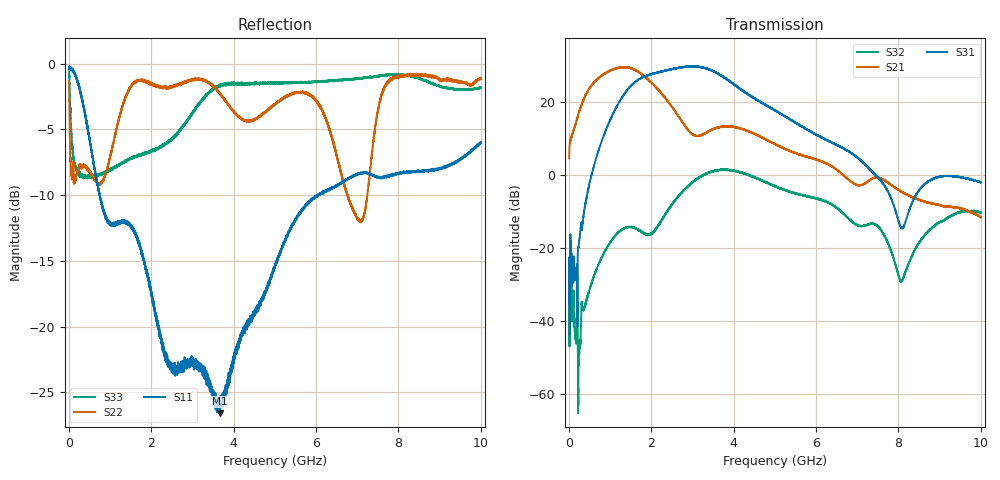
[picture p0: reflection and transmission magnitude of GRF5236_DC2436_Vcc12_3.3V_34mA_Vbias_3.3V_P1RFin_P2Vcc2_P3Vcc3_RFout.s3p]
!Keysight Technologies,N5245B,MY56052315,A.20.20.05
!Date: Friday, August 21, 2026 13:52:32
!Correction: S11(C  3-Port  )
!S12(C  3-Port  )
!S13(C  3-Port  )
!S21(C  3-Port  )
!S22(C  3-Port  )
!S23(C  3-Port  )
!S31(C  3-Port  )
!S32(C  3-Port  )
!S33(C  3-Port  )
!S3P File: Measurements: <S11,S12,S13>,
!<S21,S22,S23>,
!<S31,S32,S33>:
# Hz S  RI  R 50
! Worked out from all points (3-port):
!   9991 points, 10 MHz to 10 GHz, reference 50 ohm
!   strongest paths, dB at 10 MHz, 2.507 GHz, 5.005 GHz, 7.503 GHz, 10 GHz:
!     S31: -29.2, 29.0, 17.7, -0.8, -2.0
!     S21: 4.6, 18.6, 8.4, -0.7, -11.6
!     S32: -34.5, -8.1, -3.0, -14.1, -10.4
!   lowest |S11| = -26.6 dB at 3.659 GHz (marker M1), VSWR 1.10, Z = 51.8 + j4.4 ohm
!   |S11| at or under -10 dB: 749.2 MHz to 6.039 GHz (5.289 GHz wide, 156 % of centre); 6.039756 GHz to 6.042862 GHz (3.106 MHz wide, 0.0514 % of centre); 6.052386 GHz to 6.055565 GHz (3.178 MHz wide, 0.0525 % of centre)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
1e7  0.9557 -0.0309  0.00113 -0.000517  -9.6e-05 -0.0014
     0.4161 1.637  0.6187 -0.5937  0.00137 -0.000408
     -0.00536 -0.0343  0.0169 0.0083  0.8904 -0.3559
5.27e8  0.1273 -0.4768  -0.00216 0.00686  -0.000342 0.000473
        14.09 7.711  -0.3811 0.0668  0.00195 -0.00313
        0.8602 0.0866  0.029 0.00544  -0.3536 -0.1098
9.96e8  0.0231 -0.2456  0.00224 0.0104  -4.47e-05 0.000682
        24.2 -11.13  -0.4154 -0.1242  -0.0072 -0.0111
        3.83 -4  0.084 -0.0814  -0.3802 -0.1096
1.481e9  -0.1139 -0.2168  0.00141 0.0134  -0.000104 0.00103
         1.907 -29.32  -0.7914 -0.1475  -0.0242 0.00234
         -6.547 -14.73  -0.0298 -0.1922  -0.4173 -0.125
2.087e9  -0.1079 0.0424  0.00253 0.0187  0.000327 0.00163
         -14.98 -7.048  -0.7653 0.3057  -0.0102 0.0204
         -23.71 7.097  -0.0264 -0.1707  -0.4477 -0.1395
2.865e9  0.0512 0.0522  0.00145 0.0227  0.000504 0.00156
         -4.308 0.5593  -0.6687 0.5333  -0.00638 0.0222
         4.931 30.07  -0.4132 -0.539  -0.5716 -0.1885
3.278e9  0.0556 0.0387  0.00017 0.0269  0.000628 0.00149
         -3.47 -1.047  -0.6585 0.5582  -0.00183 0.033
         24.32 16.73  -0.9714 -0.2734  -0.7302 -0.1404
3.659e9  0.0198 0.0424  -0.000264 0.0325  0.000459 0.00188
         -4.464 -0.6976  -0.551 0.5383  0.0145 0.0381
         23.52 -3.007  -1.079 0.4385  -0.8208 0.0142
5.005e9  -0.1458 0.0836  0.00881 0.0414  0.000598 0.00231
         -1.568 2.126  -0.2773 0.6436  0.0288 0.00241
         -1.23 -7.57  0.321 0.6265  -0.8017 0.257
1e10  -0.1212 0.4866  0.0359 0.0343  0.000599 0.00131
      0.1613 0.208  -0.0982 0.8729  0.0245 0.00103
      -0.6559 0.4427  0.2912 -0.0787  0.2685 0.7655
